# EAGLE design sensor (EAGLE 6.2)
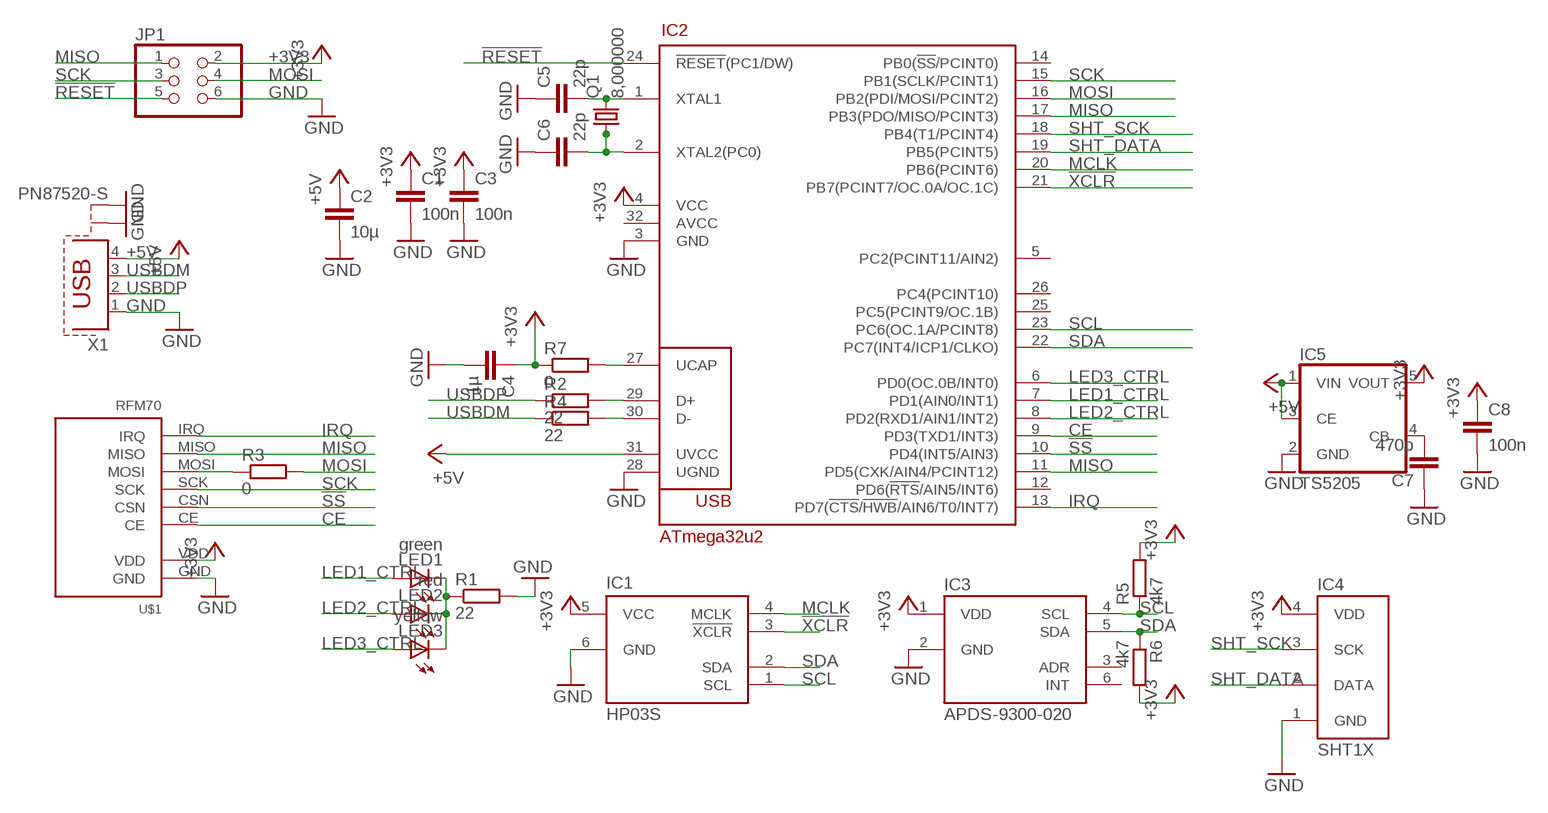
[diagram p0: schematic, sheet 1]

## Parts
C1  100n  C-EUC1206K  [C1206K]
C2  10µ  C-EUC1206K  [C1206K]
C3  100n  C-EUC1206K  [C1206K]
C4  1µ  C-EUC1206K  [C1206K]
C5  22p  C-EUC1206K  [C1206K]
C6  22p  C-EUC1206K  [C1206K]
C7  470p  C-EUC1206K  [C1206K]
C8  100n  C-EUC1206K  [C1206K]
IC1  HP03S  [HP03S]
IC2  ATmega32u2  MEGA8/16/32-2UATMEGA8/16/32U2-TQFP32  [TQFP32-08]
IC3  APDS-9300-020  APDS-9300  [APDS/SMD]
IC4  SHT1X  [SHT1X]
IC5  TS5205  [SOT25]
JP1  PINHD-2X3  [2X03]
LED1  green  LEDCHIPLED_1206  [CHIPLED_1206]
LED2  red  LEDCHIPLED_1206  [CHIPLED_1206]
LED3  yellow  LEDCHIPLED_1206  [CHIPLED_1206]
Q1  8,000000  CRYSTALHC49U-V  [HC49U-V]
R1  22  R-EU_R1206  [R1206]
R2  22  R-EU_R1206  [R1206]
R3  0  R-EU_R1206  [R1206]
R4  22  R-EU_R1206  [R1206]
R5  4k7  R-EU_R1206  [R1206]
R6  4k7  R-EU_R1206  [R1206]
R7  0  R-EU_R1206  [R1206]
U$1  RFM70  [RFM70]
X1  PN87520-S  [PN87520-S]

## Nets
!RESET: IC2.24(!RESET!(PC1/DW)) JP1.5
!SS: IC2.10(PD4(INT5/AIN3)) U$1.CSN
!XCLR: IC1.3(!XCLR) IC2.21(PB7(PCINT7/OC.0A/OC.1C))
+3V3: C1.1 C3.1 C4.1 C8.1 IC1.5(VCC) IC2.4(VCC) IC3.1(VDD) IC4.4(VDD) IC5.5(VOUT) JP1.2 R5.2 R6.2 R7.1 U$1.VDD
+5V: C2.1 IC2.31(UVCC) IC5.1(VIN) IC5.3(CE) X1.4
CE: IC2.9(PD3(TXD1/INT3)) U$1.CE
GND: C1.2 C2.2 C3.2 C4.2 C5.1 C6.1 C7.1 C8.2 IC1.6(GND) IC2.3(GND) IC2.28(UGND) IC3.2(GND) IC4.1(GND) IC5.2(GND) JP1.6 R1.2 U$1.GND X1.1 X1.S1 X1.S2
IRQ: IC2.13(PD7(!CTS!/!HWB!/AIN6/T0/INT7)) U$1.IRQ
LED1_CTRL: IC2.7(PD1(AIN0/INT1)) LED1.A
LED2_CTRL: IC2.8(PD2(RXD1/AIN1/INT2)) LED2.A
LED3_CTRL: IC2.6(PD0(OC.0B/INT0)) LED3.A
MCLK: IC1.4(MCLK) IC2.20(PB6(PCINT6))
MISO: IC2.11(PD5(CXK/AIN4/PCINT12)) IC2.17(PB3(PDO/MISO/PCINT3)) JP1.1 U$1.MISO
MOSI: IC2.16(PB2(PDI/MOSI/PCINT2)) JP1.4 R3.2
MOSI2: R3.1 U$1.MOSI
N$1: C5.2 IC2.1(XTAL1) Q1.2
N$2: C6.2 IC2.2(XTAL2(PC0)) Q1.1
N$3: IC2.29(D+) R2.2
N$4: C7.2 IC5.4(CB)
N$6: LED1.C LED2.C LED3.C R1.1
N$7: IC2.30(D-) R4.2
N$9: IC2.27(UCAP) R7.2
SCK: IC2.15(PB1(SCLK/PCINT1)) JP1.3 U$1.SCK
SCL: IC1.1(SCL) IC2.23(PC6(OC.1A/PCINT8)) IC3.4(SCL) R5.1
SDA: IC1.2(SDA) IC2.22(PC7(INT4/ICP1/CLKO)) IC3.5(SDA) R6.1
SHT_DATA: IC2.19(PB5(PCINT5)) IC4.2(DATA)
SHT_SCK: IC2.18(PB4(T1/PCINT4)) IC4.3(SCK)
USBDM: R4.1 X1.3
USBDP: R2.1 X1.2
Unconnected: IC2.5(PC2(PCINT11/AIN2)) IC2.12(PD6(!RTS!/AIN5/INT6)) IC2.14(PB0(!SS!/PCINT0)) IC2.25(PC5(PCINT9/OC.1B)) IC2.26(PC4(PCINT10)) IC2.32(AVCC) IC3.3(ADR) IC3.6(INT)

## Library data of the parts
C1-C8 = rcl:C-EU: CAPACITOR, European symbol
IC1 = pollin:HP03S: HP03S Barometer and Temperature Sensor The HP03 is a low power device, include a piezo-resistive pressure senor and an ADC interface. It provides 16 bit data for pressure and temperature relate voltage. 11 unique coefficients were stored on the chip, thus accurate pressure and temperature reading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
IC2 = avr-7:MEGA8/16/32-2U: ATmega8-2U / ATmega16-2U / ATmega32-2U 8-bit AVR Microcontroller with 8/16/32K Bytes of ISP Flash Memory and built in USB device controller
IC3 = avago:APDS-9300
IC4 = sht10_11_15:SHT1X
IC5 = v-reg:TS5205: 150mA Low Noise LDO Voltage Regulator with Enable TSC [Taiwan Semiconductor Company, Ltd] Source: http://www.taiwansemi.com .. 5205_0409c.pdf
JP1 = pinhead:PINHD-2X3: PIN HEADER
LED1-LED3 = led:LED: LED
Q1 = crystal:CRYSTAL: CRYSTAL; OC_FARNELL: 1666969; OC_NEWARK: unknown
R1-R7 = rcl:R-EU_: RESISTOR, European symbol
U$1 = rfm70:RFM70: RFM70 2.4 Ghz Funkmodul Autor: Daniel Weber Website: http://projects.web4clans.com Email: daniel.weber@web4clans.com
X1 = con-berg:PN87520-S; OC_FARNELL: unknown; OC_NEWARK: unknown

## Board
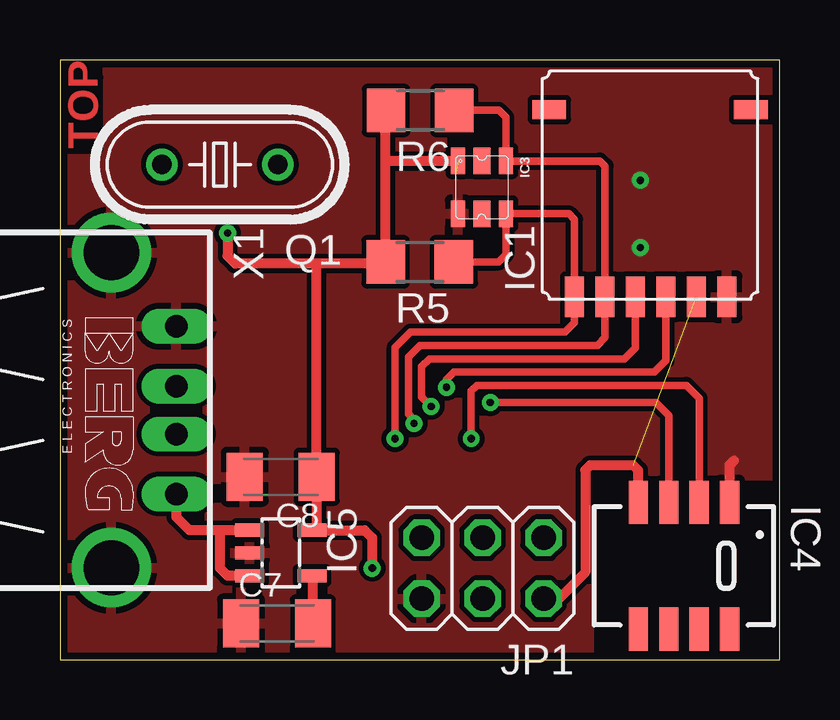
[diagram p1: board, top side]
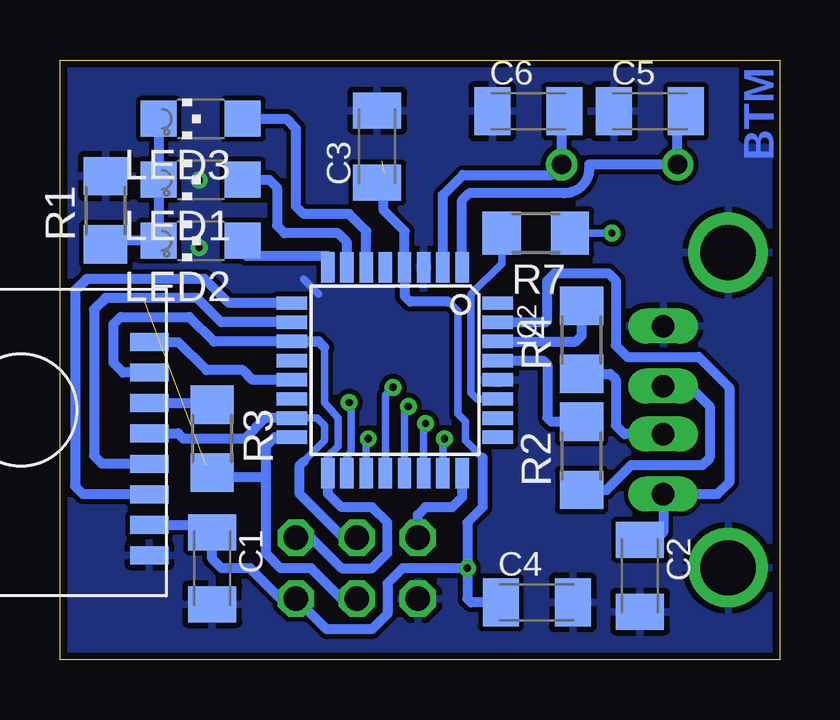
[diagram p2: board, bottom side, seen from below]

Size 30 x 25 mm. Coordinates in mm from the lower left corner, seen from the top.
Outline: 0,0 30,0 30,25 0,25 0,0
Copper layers (1*16): Top 0.035mm / dielectric 1.5mm / Bottom 0.035mm
Design rules: minimum track width 10mil, minimum drill 0.3mm, track to track 8mil, track to pad 8mil, pad to pad 8mil, via to via 8mil, smd to smd 8mil, copper to edge 12mil, drill to drill 8mil, minimum pad ring 10mil, minimum via ring 8mil, stop-mask expansion 4mil, vias tented up to drill 0mil, thermal gap 10mil

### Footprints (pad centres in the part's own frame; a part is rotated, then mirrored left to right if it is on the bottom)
C1206K = smd 1.5 x 2: 1 -1.5,0; 2 1.5,0
HP03S = smd 1.7 x 0.8: 1 -4.65,3.15; 2 -4.65,1.88; 3 -4.65,0.61; 4 -4.65,-0.66; 5 -4.65,-1.93; 6 -4.65,-3.2 | smd 0.8 x 1.4: NC@1 3.15,4.2; NC@2 3.15,-4.2
TQFP32-08 = smd 1.27 x 0.559: 1 -4.293,2.8; 2 -4.293,2; 3 -4.293,1.2; 4 -4.293,0.4; 5 -4.293,-0.4; 6 -4.293,-1.2; 7 -4.293,-2; 8 -4.293,-2.8; 17 4.293,-2.8; 18 4.293,-2; 19 4.293,-1.2; 20 4.293,-0.4; 21 4.293,0.4; 22 4.293,1.2; 23 4.293,2; 24 4.293,2.8 | smd 0.559 x 1.27: 9 -2.8,-4.293; 10 -2,-4.293; 11 -1.2,-4.293; 12 -0.4,-4.293; 13 0.4,-4.293; 14 1.2,-4.293; 15 2,-4.293; 16 2.8,-4.293; 25 2.8,4.293; 26 2,4.293; 27 1.2,4.293; 28 0.4,4.293; 29 -0.4,4.293; 30 -1.2,4.293; 31 -2,4.293; 32 -2.8,4.293
APDS/SMD = smd 1.1 x 0.6: 1 -1.1,-1; 2 1.1,-1; 4 1.1,1; 5 -1.1,1 | smd 1.1 x 0.7: 3 1.1,0; 6 -1.1,0
SHT1X = smd 1.803 x 0.8: 1 -2.642,1.905; 2 -2.642,0.635; 3 -2.642,-0.635; 4 -2.642,-1.905; 5 2.642,-1.905; 6 2.642,-0.635; 7 2.642,0.635; 8 2.642,1.905
SOT25 = smd 0.55 x 1.2: 1 -0.95,-1.3; 2 0,-1.3; 3 0.95,-1.3; 4 0.95,1.3; 5 -0.95,1.3
2X03 = drill 1.016 octagon: 1 -2.54,-1.27; 2 -2.54,1.27; 3 0,-1.27; 4 0,1.27; 5 2.54,-1.27; 6 2.54,1.27
CHIPLED_1206 = smd 1.5 x 1.5: A 0,-1.75; C 0,1.75
HC49U-V = drill 0.813: 1 -2.413,0; 2 2.413,0
R1206 = smd 1.6 x 1.803: 1 -1.422,0; 2 1.422,0
RFM70 = smd 0.75 x 1.6: CE -2.16,-7.7; CSN -0.89,-7.7; GND -4.7,-7.7; IRQ 4.19,-7.7; MISO 2.92,-7.7; MOSI 1.65,-7.7; SCK 0.38,-7.7; VDD -3.43,-7.7
PN87520-S = drill 0.95 long: 1 -3.5,2.71; 2 -1,2.71; 3 1,2.71; 4 3.5,2.71 | drill 2.3 pad 2.9: S1 -6.57,0; S2 6.57,0

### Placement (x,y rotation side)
C1  23.65,3.81 270 bottom
C2  5.82,3.49 270 bottom
C3  16.78,21.39 90 bottom
C4  10.12,2.38 0 bottom
C5  5.4,22.86 0 bottom
C6  10.48,22.86 0 bottom
C7  9.05,1.51 0 top
C8  9.21,7.62 180 top
IC1  24.6,19.77 90 top
IC2  16.03,12.06 270 bottom
IC3  17.59,19.69 270 top
IC4  26.01,3.91 270 top
IC5  9.21,4.45 270 top
JP1  17.62,3.81 180 top
LED1  24.13,20 90 bottom
LED2  24.13,17.46 90 bottom
LED3  24.13,22.54 90 bottom
Q1  6.67,20.64 180 top
R1  28.1,18.73 90 bottom
R2  8.26,8.49 90 bottom
R3  23.65,9.21 270 bottom
R4  8.26,13.34 90 bottom
R5  15,16.58 180 top
R6  15.02,22.9 180 top
R7  10.16,17.78 180 bottom
U$1  33.97,9.05 90 bottom
X1  2.14,10.4 270 top

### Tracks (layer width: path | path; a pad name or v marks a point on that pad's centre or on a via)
!RESET
  Bottom 0.406: IC2.24 13.23,6.77 13.65,6.35 14.76,6.35 15.08,6.03 JP1.5
!SS
  Bottom 0.406: IC2.10 23.27,14.06 24.29,15.08 28.1,15.08 28.57,14.61 28.57,8.49 28.24,8.16 U$1.CSN
!XCLR  (via drill 0.3)
  Top 0.305: v15.48,10.56 15.08,10.95 15.08,12.22 15.4,12.54 23.54,12.54 23.99,12.99 IC1.3
  Bottom 0.305: IC2.21 15.63,10.4 v15.48,10.56
+3V3  (via drill 0.3)  (2 unrouted)
  Top 0.406: 10.71,16.42 C8.1 10.71,5.4 10.48,5.4 10.48,5.39 IC5.5 12.7,5.39 13.02,5.08 v13.02,3.81 | IC4.4 24.11,7.89 23.9,8.1 22.1,8.1 21.9,7.9 21.9,3.64 20.8,2.54 JP1.2 | v6.99,17.78 6.99,16.83 7.3,16.51 13.51,16.51 R5.2 13.58,20.8 | 13.58,20.8 13.58,22.88 R6.2 | IC3.1 13.59,20.79 13.58,20.8
  Bottom 0.305: 13.81,14.92 13.41,14.53 13.41,10.24 13.1,9.92 13.1,9.13 12.38,8.41 | R7.1 v6.99,17.78
  Bottom 0.406: 13.81,14.92 15.4,14.92 15.63,15.16 IC2.4 15.63,17.86 16.51,18.73 16.51,20.28 16.5,20.29 C3.1 | U$1.VDD 23.65,5.62 C1.1 23.65,4.21 23.26,3.81 22.07,3.81 20.8,2.54 JP1.2 18.89,1.27 16.99,1.27 16.35,1.91 16.35,3.17 15.72,3.81 v13.02,3.81 | C4.1 12.86,2.38 13.02,2.54 v13.02,3.81 | 12.38,8.41 12.38,6.35 13.02,5.71 v13.02,3.81
+5V
  Top 0.406: IC5.1 6.67,5.39 | 6.67,5.39 5.4,5.39 4.85,5.94 X1.4 | IC5.3 6.98,3.5 6.67,3.81 6.67,5.39
  Bottom 0.406: IC2.31 9.75,14.06 9.68,14.13 9.68,15.8 9.37,16.11 7.14,16.11 6.83,15.8 6.83,13.1 6.35,12.62 3.37,12.62 2.1,11.35 2.1,7.38 2.59,6.9 X1.4 4.85,5.31 5.17,4.99 C2.1
CE
  Bottom 0.406: IC2.9 22.96,14.87 23.97,15.88 28.89,15.88 29.37,15.4 29.37,7.22 29.03,6.89 U$1.CE
GND  (via drill 0.3)
  Top 0.406: IC4.1 27.92,8.12 28.1,8.3
  Bottom 0.305: 19.21,15.24 19.84,15.88
  other vias: 24.2,19.98 24.2,17.18
  pour Bottom: 0,0 30,0 30,25 0,25
  pour Top: 0,25 30,25 30,0 0,0
IRQ
  Bottom 0.406: IC2.13 21.98,11.66 22.38,12.06 23.89,12.06 25.07,13.24 U$1.IRQ
LED1_CTRL
  Bottom 0.406: IC2.7 18.03,17.4 18.41,17.78 20.64,17.78 20.95,18.1 20.95,19.68 21.27,20 LED1.A
LED2_CTRL
  Bottom 0.406: IC2.8 18.83,16.83 22.22,16.83 LED2.A
LED3_CTRL
  Bottom 0.406: IC2.6 17.23,17.87 17.94,18.57 19.84,18.57 20.16,18.89 20.16,22.15 20.56,22.54 LED3.A
MCLK  (via drill 0.3)
  Top 0.305: v16.11,11.35 16.11,11.67 16.43,11.99 24.79,11.99 25.26,12.46 IC1.4
  Bottom 0.305: IC2.20 16.43,11.03 v16.11,11.35
MISO
  Bottom 0.305: IC2.17 18.83,8.47 18.41,8.89 18.41,10.08 18.97,10.72 18.97,13.02
  Bottom 0.406: JP1.1 19.53,5.08 18.26,3.81 16.99,3.81 16.35,4.45 16.35,5.71 16.99,6.35 18.26,6.35 18.83,6.93 IC2.17 | 18.97,13.02 19.21,13.26 | IC2.11 19.22,13.27 arc90 19.21,13.26 | 19.21,13.26 23.57,13.26 24.61,14.29 27.46,14.29 27.78,13.97 27.78,12.38 27.37,11.97 U$1.MISO
MOSI
  Bottom 0.406: JP1.4 18.26,2.54 19.53,3.81 20.8,3.81 21.43,4.45 21.43,7.62 | IC2.16 21.06,9.27 21.43,8.89 21.43,7.62 | R3.2 23.49,7.62 21.43,7.62
MOSI2
  Bottom 0.406: U$1.MOSI 23.72,10.7 R3.1
N$1
  Bottom 0.406: IC2.1 13.23,19.15 12.94,19.45 8.97,19.45 arc-90 7.94,20.48 7.94,20.64 Q1.2 4.25,22.5 C5.2
N$2
  Bottom 0.406: C6.2 9.08,22.01 Q1.1 9.52,20.2 13.2,20.2 14.03,19.37 IC2.2
N$3
  Bottom 0.406: IC2.29 9.85,12.46 9.68,12.3 9.68,10.08 9.52,9.91 R2.2
N$4
  Top 0.406: C7.2 10.55,3.45 IC5.4
N$6
  Bottom 0.406: R1.1 27.63,17.46 LED2.C LED1.C LED3.C
N$7
  Bottom 0.406: IC2.30 8.48,13.27 8.26,13.49 R4.2
N$9
  Bottom 0.305: IC2.27 12.61,10.87 12.86,11.11 12.86,15.24 11.58,16.52 R7.2
SCK
  Bottom 0.305: 19.84,8.26 18.97,9.13 18.97,9.76 19.27,10.06 IC2.15
  Bottom 0.406: JP1.3 18.18,5.08 20,6.91 20,8.1 19.84,8.26 | IC2.15 21.45,10.06 22.3,9.21 24.84,9.21 25.07,9.43 U$1.SCK
SCL  (via drill 0.3)
  Top 0.305: v13.97,9.21 13.97,13.02 14.61,13.65 21.05,13.65 21.45,14.05 IC1.1 21.45,18.35 21.21,18.59 IC3.4 18.59,16.89 18.28,16.58 R5.1
  Bottom 0.305: IC2.23 14.03,9.14 v13.97,9.21
SDA  (via drill 0.3)
  Top 0.305: v14.76,9.84 14.76,10 14.53,10.24 14.53,12.62 15,13.1 22.4,13.1 22.72,13.42 IC1.2 22.72,20.58 22.51,20.79 IC3.5 18.59,22.61 18.3,22.9 R6.1
  Bottom 0.305: IC2.22 14.83,9.61 v14.76,9.84
SHT_DATA  (via drill 0.3)
  Top 0.305: v17.14,9.21 17.14,11.19 17.38,11.43 26.11,11.43 26.65,10.89 IC4.2
  Bottom 0.305: IC2.19 17.23,9.12 v17.14,9.21
SHT_SCK  (via drill 0.3)
  Top 0.305: v17.94,10.72 24.84,10.72 25.38,10.18 IC4.3
  Bottom 0.305: IC2.18 18.03,8.48 17.86,8.65 17.86,10.64 v17.94,10.72
USBDM
  Bottom 0.406: R4.1 7.07,11.91 6.83,11.67 6.83,9.76 6.46,9.4 X1.3
USBDP
  Bottom 0.406: X1.2 3.76,11.4 2.92,10.56 2.92,8.41 3.23,8.1 6.19,8.1 7.22,7.07 R2.1

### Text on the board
Top: TOP
Bottom: BTM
